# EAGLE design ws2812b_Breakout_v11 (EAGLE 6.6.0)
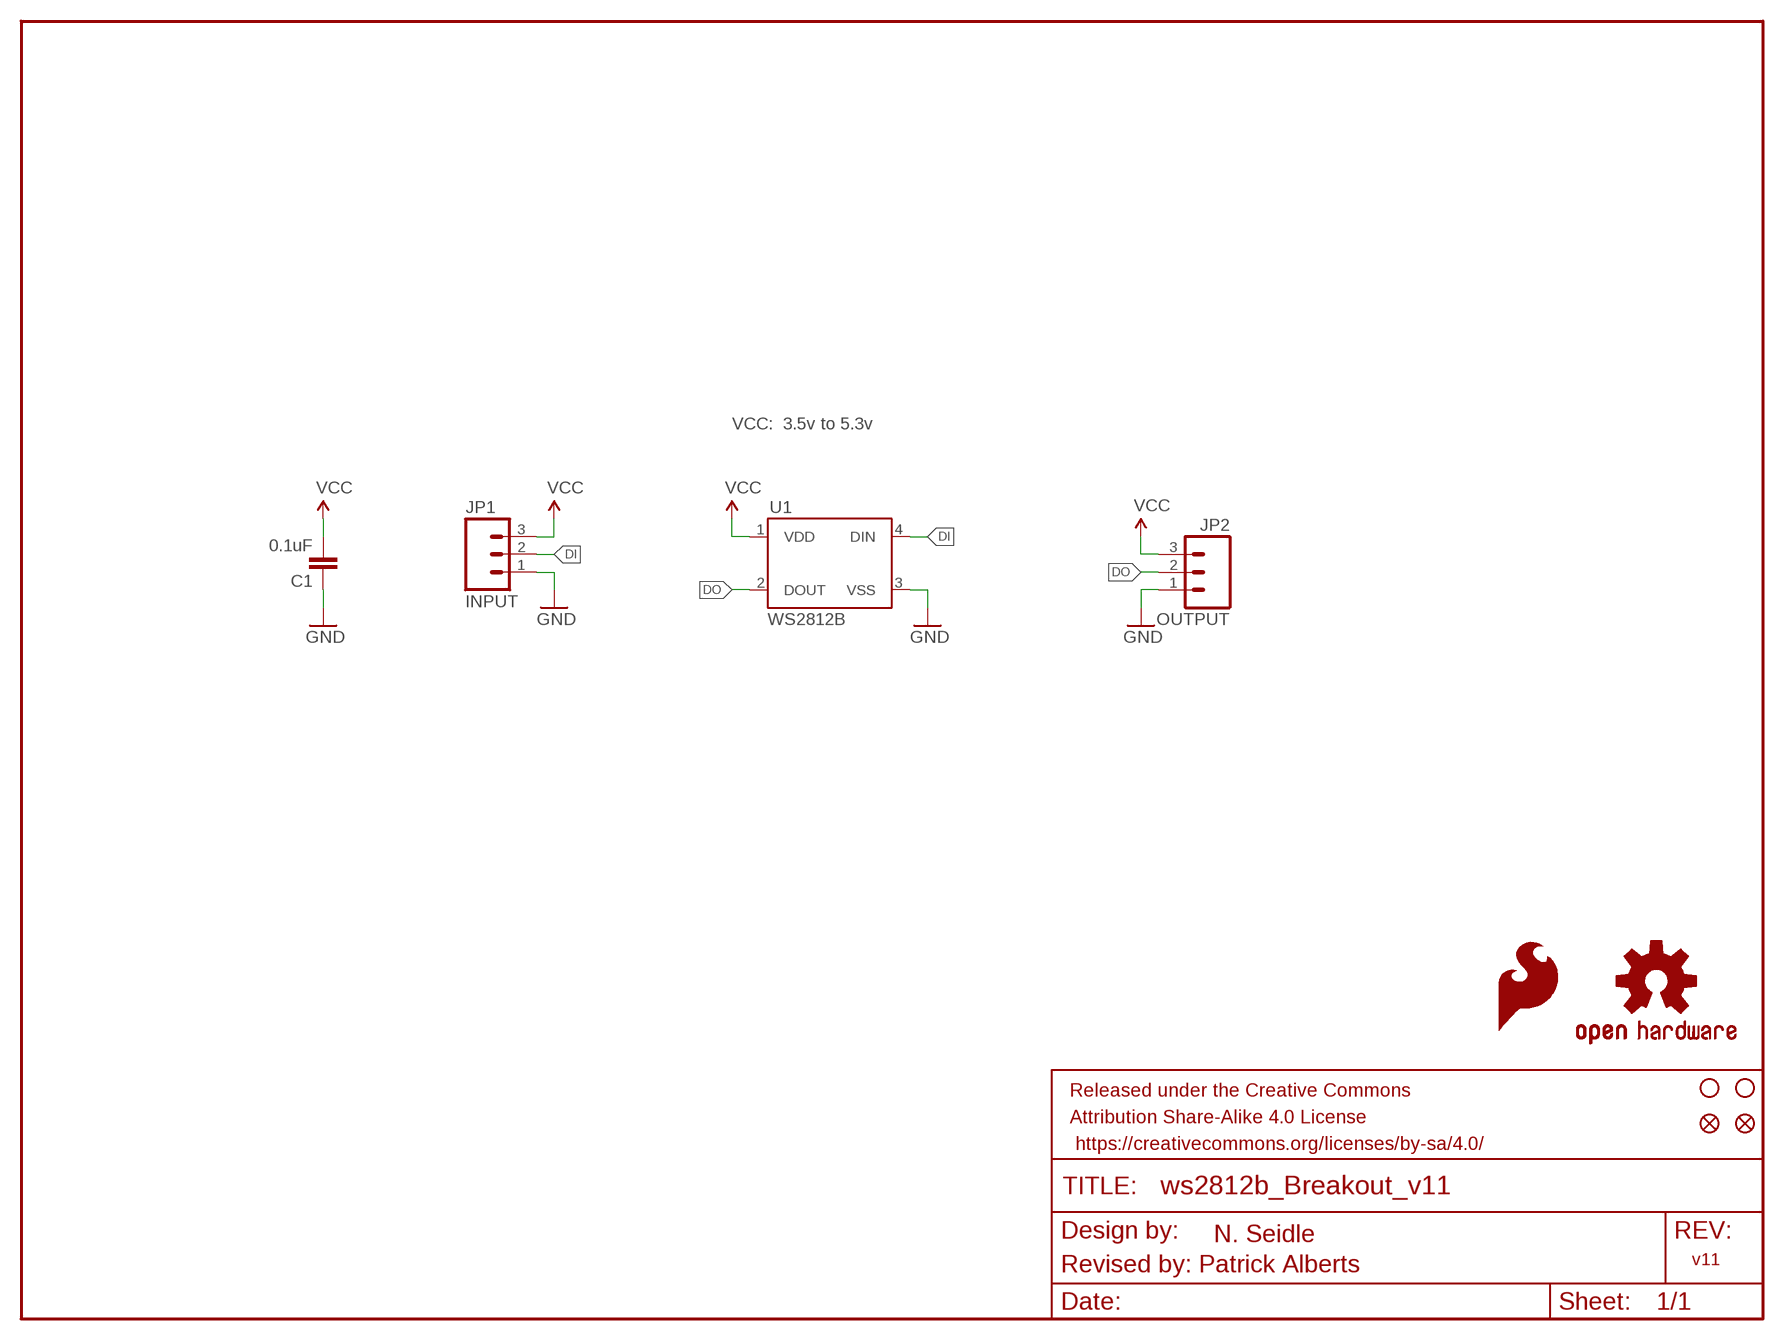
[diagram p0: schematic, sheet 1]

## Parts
C1  0.1uF  0.1UF-25V(+80/-20%)(0603)  [0603-CAP]
FID1  FIDUCIAL1X2  [FIDUCIAL-1X2]
FID2  FIDUCIAL1X2  [FIDUCIAL-1X2]
FRAME1  FRAME-LETTER  [CREATIVE_COMMONS]
JP1  INPUT  M03PTH  [1X03]
JP2  OUTPUT  M03PTH  [1X03]
JP4  STAND-OFF  [STAND-OFF]
JP15  STAND-OFF  [STAND-OFF]
LOGO1  OSHW-LOGOS  [OSHW-LOGO-S]
LOGO2  SFE_LOGO_FLAME.1_INCH  [SFE_LOGO_FLAME_.1]
U1  WS2812B  [WS2812B]

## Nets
DI: JP1.2 U1.4(DIN)
DO: JP2.2 U1.2(DOUT)
GND: C1.1 JP1.1 JP2.1 U1.3(VSS)
VCC: C1.2 JP1.3 JP2.3 U1.1(VDD)

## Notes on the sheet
- VCC:  3.5v to 5.3v
- N. Seidle
- v11
- Revised by: Patrick Alberts

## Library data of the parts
C1 = SparkFun-Capacitors:0.1UF-25V(+80/-20%)(0603): CAP-00810; PROD_ID: CAP-00810
FID1 FID2 = SparkFun-Aesthetics:FIDUCIAL: Fiducial Alignment Points
FRAME1 = SparkFun-Aesthetics:FRAME-LETTER: Schematic Frame; DESIGNER: NAME; VERSION: v01
JP1 JP2 = SparkFun-Connectors:M03: Header 3 Standard 3-pin 0.1" header. Use with straight break away headers (SKU : PRT-00116), right angle break away headers (PRT-00553), swiss pins (PRT-00743), machine pins (PRT-00117), and female headers (PRT-00115). Molex polarized connector foot print use with SKU : PRT-08232 with associated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
JP4 JP15 = SparkFun:STAND-OFF: Stand Off
LOGO1 = SparkFun-Aesthetics:OSHW-LOGO: Open Source Hardware Logo
LOGO2 = SparkFun-Aesthetics:SFE_LOGO_FLAME: SFE Logo, flame only
U1 = SparkFun-LED:WS2812B: WS2812B - Intelligent control LED integrated light source Technical Specifications: Power Supply Voltage (VDD): 3.5 to 5.3 V Input Voltage (VI): -0.5 to VDD+0.5 V Operating Junction Temperature (Topt): -25°C to +80°C Storage Temperature Range (Tstg): -55°C to +150°C; PROD_ID: DIO-12503

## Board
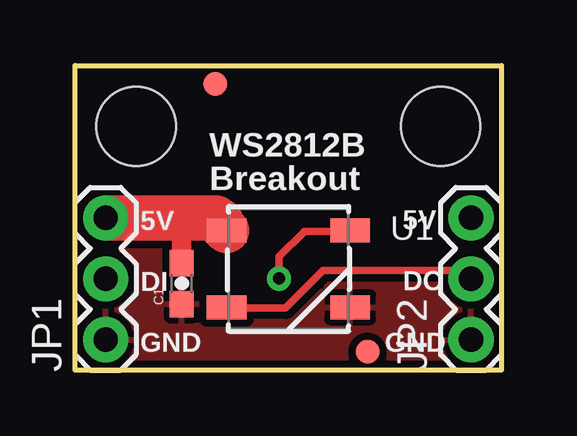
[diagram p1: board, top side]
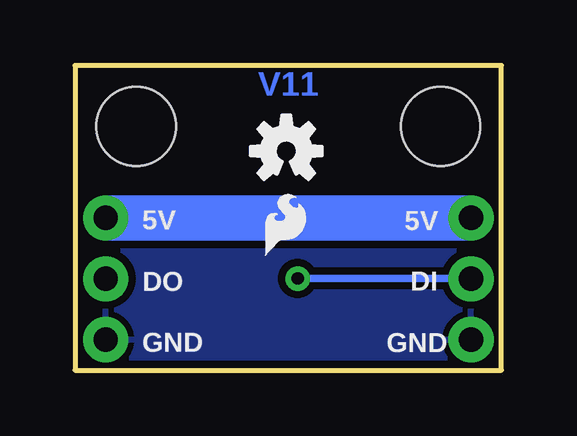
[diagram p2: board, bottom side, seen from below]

Size 17.78 x 12.7 mm. Coordinates in mm from the lower left corner, seen from the top.
Outline: 0,0 0,12.7 17.78,12.7 17.78,0 0,0
Copper layers (1*16): Top 0.035mm / dielectric 1.5mm / Bottom 0.035mm
Design rules "SparkFun-2-layer": minimum track width 7mil, minimum drill 15mil, track to track 8mil, track to pad 8mil, pad to pad 8mil, via to via 8mil, smd to smd 8mil, copper to edge 8mil, drill to drill 8mil, minimum pad ring 12mil, minimum via ring 10mil, stop-mask expansion 4mil, vias tented up to drill 20mil, thermal gap 10mil

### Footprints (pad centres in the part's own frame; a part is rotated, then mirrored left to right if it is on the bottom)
0603-CAP = smd 1.1 x 1: 1 -0.85,0; 2 0.85,0
FIDUCIAL-1X2 = smd 1 x 1: 1 0,0
1X03 = drill 1.016 pad 1.88: 1 0,0; 2 2.54,0; 3 5.08,0
STAND-OFF = hole 3.302: 0,0
WS2812B = smd 1.651 x 1: 1 -2.577,1.6; 2 -2.577,-1.6; 3 2.577,-1.6; 4 2.577,1.6

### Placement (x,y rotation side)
C1  4.45,3.61 90 top
FID1  5.84,11.94 0 top
FID2  12.19,0.76 0 top
FRAME1  not placed on the board
JP1  1.27,1.27 90 top
JP2  16.51,1.27 90 top
JP4  2.54,10.16 0 top
JP15  15.24,10.16 0 top
LOGO1  8.98,9.14 0 bottom
LOGO2  10.16,4.44 0 bottom
U1  8.89,4.22 0 top

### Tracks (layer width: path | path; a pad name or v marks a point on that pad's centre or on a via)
DI  (via drill 0.51)
  Top 0.305: v8.5,3.82 8.5,4.73 9.56,5.79 11.44,5.79 U1.4
  Bottom 0.305: JP1.2 v8.5,3.82
DO
  Top 0.305: JP2.2 16.17,4.15 10.34,4.15 8.78,2.59 6.34,2.59 U1.2
GND
  pour Top (isolate 0.305): 0,7.62 0,0 17.78,0 17.78,7.62
  pour Bottom (isolate 0.305): 0,7.62 0,0 17.78,0 17.78,7.62
VCC
  Top 0.813: 4.57,5.97 4.7,5.97 | 4.7,5.97 5.08,6.35 | C1.2 4.45,5.71 4.7,5.97
  Top 1.905: JP1.3 5.08,6.35 5.88,6.35 5.88,6.22 6.06,6.22 6.06,6.07 U1.1
  Bottom 1.905: JP2.3 JP1.3

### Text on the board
Bottom: V11
tPlace: WS2812B | Breakout | 5V | 5V | DI | DO | GND | GND
bPlace: 5V | 5V | DI | DO | GND | GND
Document: N. Seidle
tDocu: N. Seidle | Revised by: Patrick Alberts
